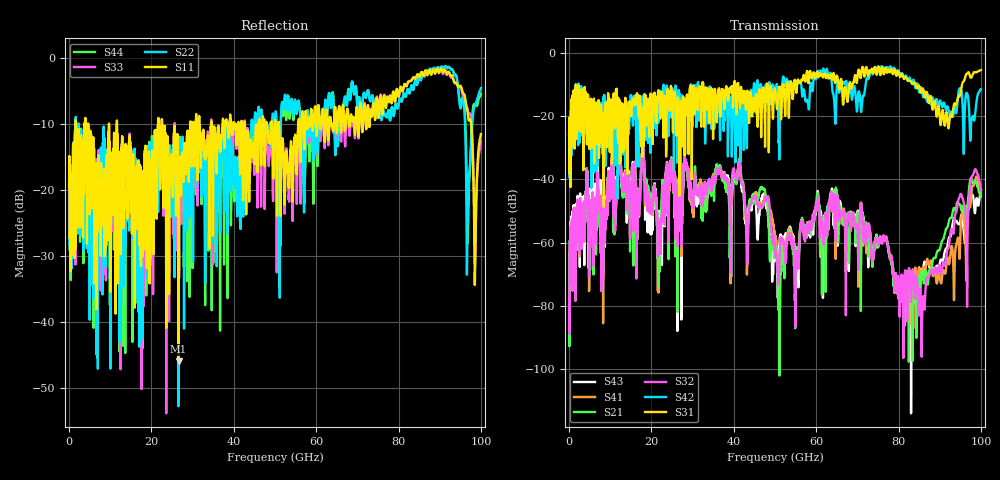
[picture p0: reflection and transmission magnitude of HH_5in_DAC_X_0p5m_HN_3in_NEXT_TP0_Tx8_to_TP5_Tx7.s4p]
# GHz S RI R 45
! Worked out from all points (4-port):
!   4000 points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, 25 MHz to 100 GHz, reference 45 ohm
!   strongest paths, dB at 25 MHz, 25.02 GHz, 50.02 GHz, 75.03 GHz, 100 GHz:
!     S31: -25.9, -17.6, -11.9, -4.7, -5.4
!     S42: -26.1, -11.5, -14.7, -4.3, -11.5
!     S32: -79.5, -34.6, -63.2, -59.6, -43.4
!     S21: -81.0, -34.4, -64.4, -60.7, -45.6
!     S41: -79.5, -34.9, -58.9, -60.2, -43.4
!     S43: -77.6, -35.0, -63.2, -61.1, -43.5
!   lowest |S11| = -46.0 dB at 26.6 GHz (marker M1), VSWR 1.01, Z = 44.6 - j0.0514 ohm
!   |S11| at or under -10 dB: 4.661 GHz to 9.697 GHz (5.036 GHz wide, 70.1 % of centre); 11.65 GHz to 21.63 GHz (9.977 GHz wide, 60 % of centre); 22.59 GHz to 29.47 GHz (6.872 GHz wide, 26.4 % of centre)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
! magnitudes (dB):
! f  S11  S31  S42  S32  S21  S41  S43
! 25 MHz  -19.4  -25.9  -26.1  -79.5  -81.0  -79.5  -77.6
! 12.22 GHz  -16.5  -16.2  -22.1  -30.5  -31.2  -29.8  -29.1
! 26.6 GHz  -46.0  -16.5  -12.8  -47.4  -46.6  -44.4  -45.4
! 51.05 GHz  -11.1  -10.8  -33.7  -67.7  -88.8  -75.7  -61.3
! 64.05 GHz  -10.6  -7.3  -12.5  -49.2  -44.2  -45.6  -46.4
! 85.92 GHz  -2.5  -11.3  -13.9  -77.8  -70.2  -67.8  -68.4
! 100 GHz  -11.5  -5.4  -11.5  -43.4  -45.6  -43.4  -43.5
